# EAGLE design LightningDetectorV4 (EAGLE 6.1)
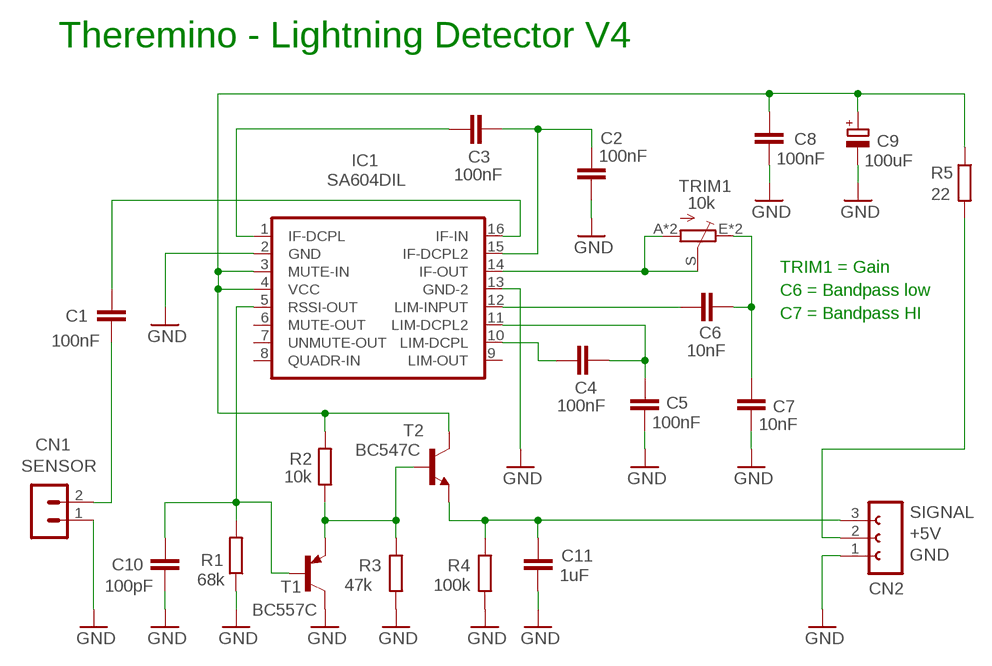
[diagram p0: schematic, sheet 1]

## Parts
C1  100nF  C-EU050-024X044  [C050-024X044]
C2  100nF  C-EU050-024X044  [C050-024X044]
C3  100nF  C-EU050-024X044  [C050-024X044]
C4  100nF  C-EU050-024X044  [C050-024X044]
C5  100nF  C-EU050-024X044  [C050-024X044]
C6  10nF  C-EU050-024X044  [C050-024X044]
C7  10nF  C-EU050-024X044  [C050-024X044]
C8  100nF  C-EU050-024X044  [C050-024X044]
C9  100uF  CPOL-EUE2-5B  [E2-5B]
C10  100pF  C-EU050-024X044  [C050-024X044]
C11  1uF  C-EU050-024X044  [C050-024X044]
CN1  SENSOR  MA02-1L2  [MA02-1_L2]
CN2  OUT  FE03-1"  [FE03-1]
IC1  SA604DIL  [DIL16]
R1  68k  R-EU_0204/7  [0204/7]
R2  10k  R-EU_0204/7  [0204/7]
R3  47k  R-EU_0204/7  [0204/7]
R4  100k  R-EU_0204/7  [0204/7]
R5  22  R-EU_0204/7  [0204/7]
T1  BC557C  -PNP-TO92-CBE  [TO92-CBE]
T2  BC547C  -NPN-TO92-CBE  [TO92-CBE]
TRIM1  10k  TRIMMERTRIM_1H  [TRIM_1H]

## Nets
GND: C2.1 C5.1 C7.1 C8.2 C9.- C10.1 C11.1 CN1.1 CN2.1 IC1.2(GND) IC1.13(GND-2) R1.1 R3.1 R4.1 T1.C
N$1: C8.1 C9.+ IC1.3(MUTE-IN) IC1.4(VCC) R2.2 R5.1 T2.C
N$2: C4.2 C5.2 IC1.11(LIM-DCPL2)
N$3: C4.1 IC1.10(LIM-DCPL)
N$4: CN2.2 R5.2
N$5: C6.1 IC1.12(LIM-INPUT)
N$6: IC1.14(IF-OUT) TRIM1.A TRIM1.A2(A) TRIM1.S
N$8: C6.2 C7.2 TRIM1.E TRIM1.E2(E)
N$9: C2.2 C3.2 IC1.15(IF-DCPL2)
N$10: C3.1 IC1.1(IF-DCPL)
N$11: C1.2 IC1.16(IF-IN)
N$13: C10.2 IC1.5(RSSI-OUT) R1.2 T1.B
N$14: R2.1 R3.2 T1.E T2.B
N$15: C11.2 CN2.3 R4.2 T2.E
N$16: C1.1 CN1.2
Unconnected: IC1.6(MUTE-OUT) IC1.7(UNMUTE-OUT) IC1.8(QUADR-IN) IC1.9(LIM-OUT)

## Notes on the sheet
- Theremino - Lightning Detector V4
- TRIM1 = Gain
- C6 = Bandpass low
- C7 = Bandpass HI
- SIGNAL
- +5V
- GND

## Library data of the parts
C1-C8 C10 C11 = 00-LIVIO:C-EU: CAPACITOR, European symbol
C9 = 00-LIVIO:CPOL-EU: POLARIZED CAPACITOR, European symbol
CN1 = 03-con-lstb-M:MA02-1: PIN HEADER
CN2 = 02-con-lsta-F:FE03-1: FEMALE HEADER
IC1 = 00-LIVIO:SA604: High-performance low-power FM IF system
R1-R5 = 00-LIVIO:R-EU_: RESISTOR, European symbol
T1 = 00-LIVIO:*-PNP-: PNP Transistror
T2 = 00-LIVIO:*-NPN-: NPN Transistror
TRIM1 = 00-LIVIO:TRIMMER: Horizzontal and Vertical trimmers

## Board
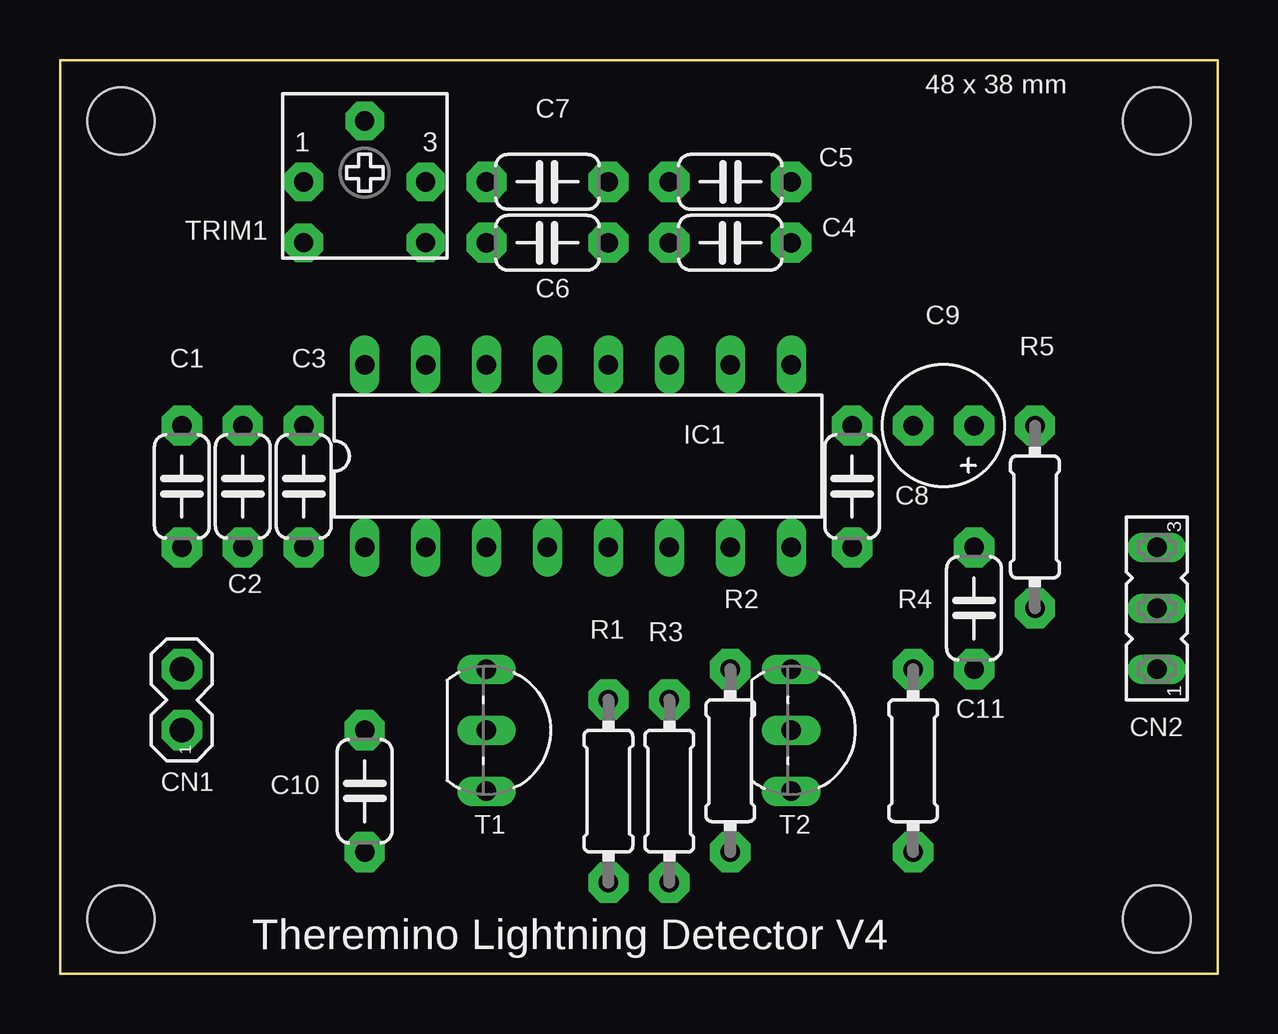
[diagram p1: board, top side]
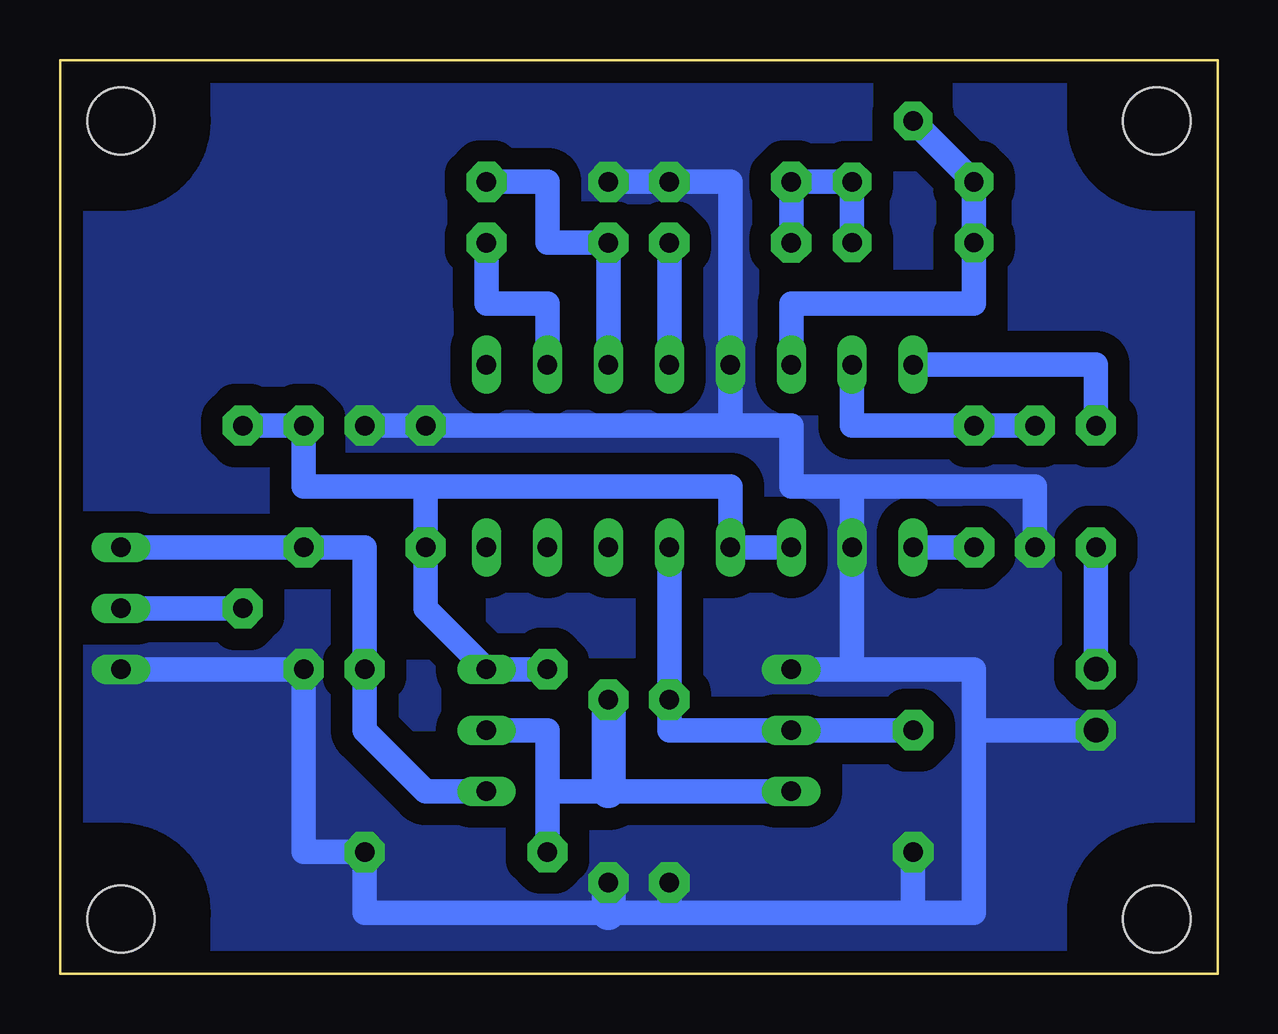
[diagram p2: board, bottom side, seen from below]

Size 48.26 x 38.1 mm. Coordinates in mm from the lower left corner, seen from the top.
Outline: 0,0 48.26,0 48.26,38.1 0,38.1 0,0
Copper layers (1*16): Top 0.035mm / dielectric 1.5mm / Bottom 0.035mm
Design rules: minimum track width 10mil, minimum drill 0.6mm, track to track 8mil, track to pad 8mil, pad to pad 8mil, via to via 8mil, smd to smd 8mil, copper to edge 31mil, drill to drill 8mil, minimum pad ring 5mil, minimum via ring 8mil, stop-mask expansion 4mil, vias tented up to drill 0mil, thermal gap 47mil
Holes 2.8 mm at 2.54,35.56 45.72,35.56 45.72,2.29 2.54,2.29
bRestrict: 12 lines

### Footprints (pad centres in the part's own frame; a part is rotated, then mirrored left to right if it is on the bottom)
C050-024X044 = drill 0.813 pad 1.676 octagon: 1 -2.54,0; 2 2.54,0
E2-5B = drill 0.813 pad 1.676 octagon: + -1.27,0; - 1.27,0
MA02-1_L2 = drill 1.016 pad 1.676 octagon: 1 -1.27,0; 2 1.27,0
FE03-1 = drill 0.813 long: 1 -2.54,0; 2 0,0; 3 2.54,0
DIL16 = drill 0.813 long: 1 -8.89,-3.81; 2 -6.35,-3.81; 3 -3.81,-3.81; 4 -1.27,-3.81; 5 1.27,-3.81; 6 3.81,-3.81; 7 6.35,-3.81; 8 8.89,-3.81; 9 8.89,3.81; 10 6.35,3.81; 11 3.81,3.81; 12 1.27,3.81; 13 -1.27,3.81; 14 -3.81,3.81; 15 -6.35,3.81; 16 -8.89,3.81
0204/7 = drill 0.813 pad 1.676 octagon: 1 -3.81,0; 2 3.81,0
TO92-CBE = drill 0.813 long: B 0,0; C -2.54,0; E 2.54,0
TRIM_1H = drill 0.8 pad 1.6 octagon: A -2.54,0; A2 -2.54,-2.54; E 2.54,0; E2 2.54,-2.54; S 0,2.54

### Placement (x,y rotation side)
C1  5.08,20.32 90 top
C2  7.62,20.32 90 top
C3  10.16,20.32 90 top
C4  27.94,30.48 180 top
C5  27.94,33.02 0 top
C6  20.32,30.48 180 top
C7  20.32,33.02 180 top
C8  33.02,20.32 90 top
C9  36.83,22.86 180 top
C10  12.7,7.62 90 top
C11  38.1,15.24 90 top
CN1  5.08,11.43 90 top
CN2  45.72,15.24 90 top
IC1  21.59,21.59 0 top
R1  22.86,7.62 90 top
R2  27.94,8.89 90 top
R3  25.4,7.62 90 top
R4  35.56,8.89 90 top
R5  40.64,19.05 270 top
T1  17.78,10.16 270 top
T2  30.48,10.16 270 top
TRIM1  12.7,33.02 0 top

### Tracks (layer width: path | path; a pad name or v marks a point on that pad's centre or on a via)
GND
  Bottom 1.016: 22.86,2.54 25.4,2.54 35.56,2.54 R4.1 38.1,5.08 C11.1 CN2.1 | 22.86,2.54 12.7,2.54 | 12.7,2.54 10.16,2.54 10.16,10.16 | R1.1 22.86,2.54 | C5.1 C7.1 20.32,33.02 IC1.13 20.32,22.86 | 15.24,20.32 IC1.2 15.24,12.7 | 15.24,20.32 17.78,20.32 17.78,22.86 20.32,22.86 | 20.32,22.86 C8.2 C9.- | C2.1 7.62,20.32 15.24,20.32 | 10.16,10.16 10.16,12.7 15.24,12.7 | 15.24,12.7 T1.C | CN1.1 10.16,10.16 | C10.1 12.7,2.54
  Bottom 1.422: R3.1 25.4,2.54
  pour Bottom (isolate 0.9, rank 6, no thermals): -1,-1 49.26,-1 49.26,39.1 -1,39.1
N$1
  Bottom 1.016: IC1.3 IC1.4 20.32,20.32 33.02,20.32 | R2.2 T2.C 33.02,15.24 C8.1 33.02,20.32 | 33.02,20.32 38.1,20.32 C9.+ R5.1
N$2
  Bottom 1.016: C5.2 27.94,33.02 27.94,30.48 C4.2 IC1.11
N$3
  Bottom 1.016: IC1.10 27.94,27.94 30.48,27.94 C4.1
N$4
  Bottom 1.016: CN2.2 R5.2
N$5
  Bottom 1.016: C6.1 IC1.12
N$6
  Bottom 1.016: IC1.14 17.78,27.94 10.16,27.94 TRIM1.A2 TRIM1.A TRIM1.S
N$8
  Bottom 1.016: C6.2 C7.2 TRIM1.E TRIM1.E2
N$9
  Bottom 1.016: IC1.15 15.24,22.86 C3.2 | 8.89,22.86 C3.2 | C2.2 C3.2
N$10
  Bottom 1.016: IC1.1 C3.1
N$11
  Bottom 1.016: IC1.16 5.08,25.4 C1.2
N$13
  Bottom 1.016: IC1.5 R1.2 22.86,10.16 T1.B C10.2
N$14
  Bottom 1.016: T1.E 25.4,7.62 27.94,7.62 | 27.94,7.62 27.94,10.16 T2.B | R2.1 27.94,7.62
  Bottom 1.422: R3.2 25.4,7.62
N$15
  Bottom 1.016: CN2.3 C11.2 35.56,17.78 R4.2 35.56,10.16 33.02,7.62 T2.E
N$16
  Bottom 1.016: CN1.2 C1.1

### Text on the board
tNames: 48 x 38 mm | Theremino Lightning Detector V4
